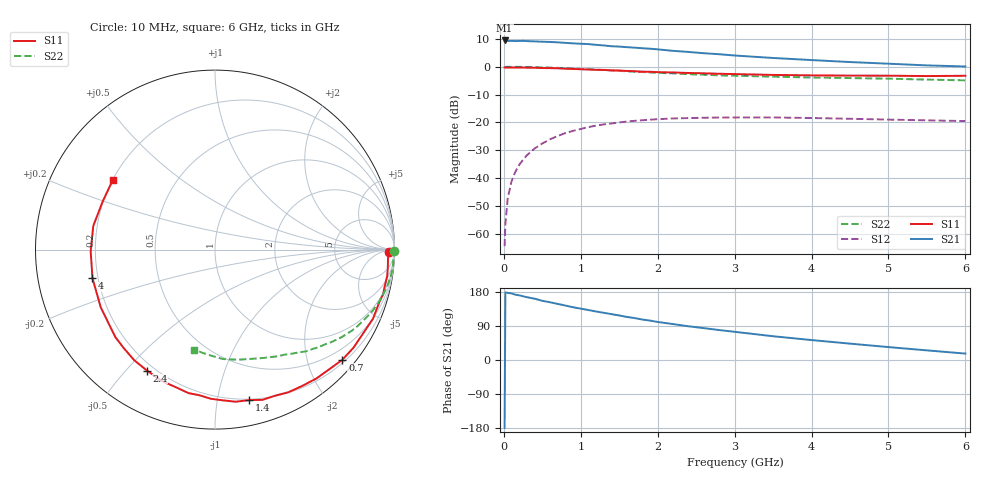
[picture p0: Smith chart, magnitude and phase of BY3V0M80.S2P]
! SIEMENS Small Signal Semiconductors
! BFY420
! Si NPN RF SIEGET Grounded Emitter Transistor in MICRO-X
! VCE = 3 V  IC = 0.8 mA
! Common Emitter S-Parameters:  October  1996
# GHz  S  MA  R  50
!  f  S11  S21  S12  S22
! GHz  MAG  ANG  MAG  ANG  MAG  ANG  MAG  ANG
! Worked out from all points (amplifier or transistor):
!   36 points, 10 MHz to 6 GHz, reference 50 ohm
!   highest |S21| = 9.4 dB at 10 MHz (marker M1)
!   |S21| within 3 dB of that: start of sweep to 1.917 GHz
!   unconditionally stable (mu >= 1): 4.638 GHz to end of sweep
!   at 250 MHz: K = 0.02, MSG = 21.4 dB, |S12| = -33.4 dB
!   at 1.4 GHz: K = 0.18, MSG = 13.9 dB, |S12| = -20.4 dB
!   at 6 GHz: K = 1.37, MAG = 6.2 dB, |S12| = -19.5 dB
!   S11 on the Smith chart (normalised r, x): 10 MHz: 55, -25; 700 MHz: 0.26, -2.67; 1.4 GHz: 0.19, -1.23; 2.4 GHz: 0.17, -0.57; 4 GHz: 0.18, -0.11; 6 GHz: 0.20, +0.30
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0.01  0.9703 -0.8  2.967 -179.4  0.0006 85.4  0.9992 -0.3
0.02  0.9668 -1.2  2.945 178.7  0.0015 94.2  0.9908 -0.5
0.05  0.9652 -3.0  2.902 177.1  0.0043 84.1  0.9983 -1.3
0.1  0.9682 -6.0  2.915 175.7  0.0088 87.9  0.9954 -2.7
0.15  0.9707 -8.8  2.892 172.3  0.013 83.4  0.9955 -4.2
0.25  0.969 -14.9  2.918 168.2  0.0213 81.3  0.9928 -6.9
0.4  0.9609 -23.6  2.857 161.8  0.034 75.9  0.9841 -11.0
0.5  0.9485 -29.4  2.818 156.2  0.0419 72.1  0.975 -13.6
0.7  0.9383 -40.8  2.745 148.0  0.0571 65.6  0.9543 -18.8
0.9  0.9137 -51.8  2.632 139.2  0.0707 58.2  0.9278 -23.6
1.1  0.8939 -62.7  2.553 131.8  0.0824 52.4  0.901 -28.3
1.4  0.8598 -77.3  2.335 121.0  0.0958 43.8  0.8591 -34.5
1.6  0.841 -87.0  2.248 113.6  0.1038 38.4  0.8289 -38.4
1.8  0.816 -96.2  2.152 106.8  0.1094 33.7  0.8027 -41.7
2.2  0.7893 -112.1  1.931 94.7  0.118 25.1  0.7604 -48.2
2.4  0.7732 -119.4  1.845 89.0  0.1198 21.8  0.7355 -51.3
2.8  0.7483 -132.7  1.679 79.0  0.1225 15.3  0.7011 -56.7
3.5  0.7132 -153.2  1.438 62.7  0.123 6.9  0.6637 -65.3
4  0.7009 -166.9  1.319 52.6  0.1201 2.6  0.6414 -71.7
4.5  0.6927 -179.2  1.215 43.2  0.1165 -0.8  0.6265 -78.3
5.5  0.6808 156.7  1.058 25.4  0.1092 -3.3  0.5878 -93.4
6  0.6888 145.7  1.011 16.9  0.1058 -2.4  0.5701 -101.9
